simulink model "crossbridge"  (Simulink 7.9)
settings: Solver=ode1  StartTime=0.0  StopTime=dt*klokmax  FixedStep=dt  RelTol=1e-3
PreLoadFcn:
  | %This Model has been adapted from the MATLAB code presented in Hoppensteadt
  | %and Peskin "Modling and Simulation in Medicine and the Life Sciences
  | 
  | %Constants for p(x)
  | p1=4;                       %units: pN
  | GAMMA=0.322;                %units: /nm
  | 
  | %Constants for u
  | alpha=14;                   %probability per unit time for attachment: /s
  | beta=126;                   %probability per unit time for detachment: /s
  | n0=10000;                   %number of crossbridges
  | A=5;                        %displacement of newly attached crossbridge: nm
  | dt=0.01/(alpha+beta);       %duration of time step: s
  | klokmax = 4000;
  | 
  | %number of bins for population density function:
  | nbins=round(sqrt(n0*alpha/(alpha+beta)));
  | 
  | %Model parameters
  | Tstart=14/(alpha+beta);    %time at which motion begins: s
  | V=500;                     %shortening velocity for t>Tstart: nm/s
  | 
  | %All crossbridges are initially detached.
  | a=zeros(1,n0);
  | x0=zeros(1,n0);
undefined symbols (not defined in the file or in its folder): randi
libraries: simulink x2

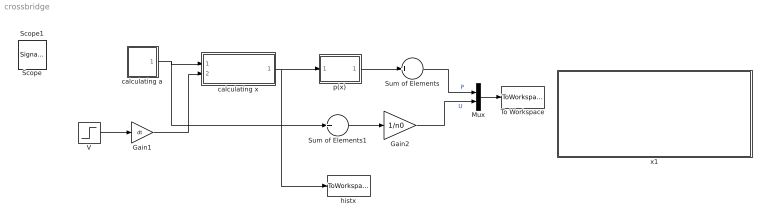
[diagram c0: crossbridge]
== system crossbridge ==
  Gain1 : Gain  Gain=dt
  Gain2 : Gain  Gain=1/n0
  Mux : Mux  Inputs=2
  Sum of Elements : Sum  Inputs=+
  Sum of Elements1 : Sum  Inputs=+
  To Workspace : ToWorkspace  VariableName=P_U  SampleTime=-1  SaveFormat=Structure With Time
  V : Step  Time=Tstart  After=V  SampleTime=0
  calculating a : Subsystem
  calculating x : Subsystem
  histx : ToWorkspace  VariableName=xout  SampleTime=-1
  p(x) : Subsystem
  x1 : Subsystem
  Scope : SignalViewerScope  IOType=viewer  RefreshTime=0.035000
  Scope1 : SignalViewerScope  IOType=viewer  RefreshTime=0.035000
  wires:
  V/1 -> Gain1/1
  calculating a/1(a) -> Sum of Elements1/1, calculating x/1(a)
  Sum of Elements1/1 -> Gain2/1
  Gain1/1 -> calculating x/2(V*dt)
  calculating x/1(calcx) -> histx/1, p(x)/1(calcx)
  Sum of Elements/1 -> Mux/1  "P"
  Gain2/1 -> Mux/2  "U"
  p(x)/1(p) -> Sum of Elements/1
  Mux/1 -> To Workspace/1

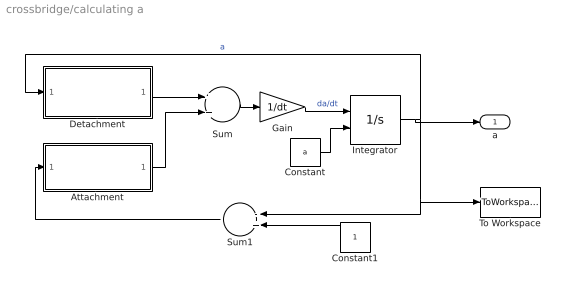
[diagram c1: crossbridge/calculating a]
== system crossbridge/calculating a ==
  Attachment : Subsystem
  Constant : Constant  Value=a
  Constant1 : Constant
  Detachment : Subsystem
  Gain : Gain  Gain=1/dt
  Integrator : Integrator  InitialConditionSource=external
  Sum : Sum
  Sum1 : Sum  Inputs=-+
  To Workspace : ToWorkspace  VariableName=aout  SampleTime=-1
  a : Outport
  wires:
  Integrator/1 -> Detachment/1(a), Sum1/1, To Workspace/1, a/1  "a"
  Constant/1 -> Integrator/2
  Detachment/1(OutD) -> Sum/1
  Attachment/1(OutA) -> Sum/2
  Sum/1 -> Gain/1
  Sum1/1 -> Attachment/1(1-a)
  Constant1/1 -> Sum1/2
  Gain/1 -> Integrator/1  "da/dt"

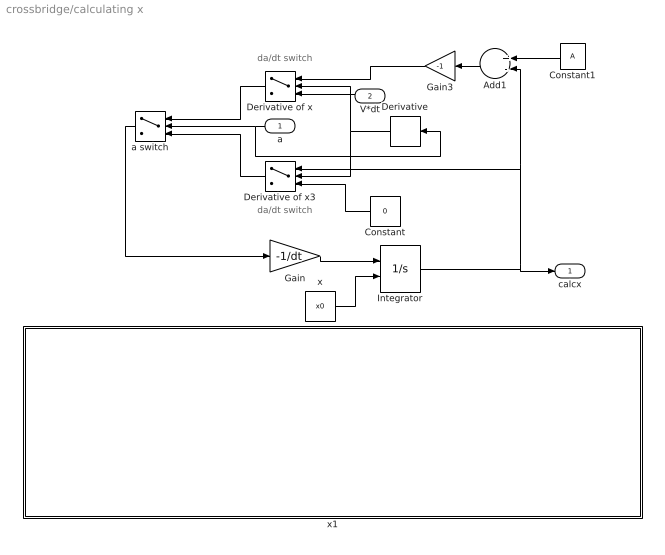
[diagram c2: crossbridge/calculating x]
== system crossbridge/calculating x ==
  note: da/dt switch
  note: da/dt switch
  a : Inport
  V*dt : Inport  Port=2
  Add1 : Sum  Inputs=+-
  Constant : Constant  Value=0
  Constant1 : Constant  Value=A
  Derivative : Derivative
  Derivative of x : Switch  Criteria=u2 ~= 0  ZeroCross=off
  Derivative of x3 : Switch  Criteria=u2 ~= 0  ZeroCross=off
  Gain : Gain  Gain=-1/dt
  Gain3 : Gain  Gain=-1
  Integrator : Integrator  InitialConditionSource=external
  a switch : Switch  Criteria=u2 ~= 0  ZeroCross=off
  x : Constant  Value=x0
  x1 : Subsystem
  calcx : Outport
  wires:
  Gain/1 -> Integrator/1
  Integrator/1 -> calcx/1, Add1/2, Derivative of x3/1
  x/1 -> Integrator/2
  Constant1/1 -> Add1/1
  Add1/1 -> Gain3/1
  Derivative/1 -> Derivative of x3/2, Derivative of x/2
  Derivative of x/1 -> a switch/1
  Derivative of x3/1 -> a switch/3
  a/1 -> a switch/2, Derivative/1
  a switch/1 -> Gain/1
  Constant/1 -> Derivative of x3/3
  V*dt/1 -> Derivative of x/3
  Gain3/1 -> Derivative of x/1

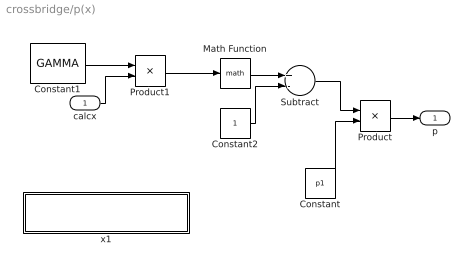
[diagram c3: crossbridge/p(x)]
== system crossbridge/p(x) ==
  calcx : Inport
  Constant : Constant  Value=p1
  Constant1 : Constant  Value=GAMMA
  Constant2 : Constant
  Math Function : Math
  Product : Product
  Product1 : Product
  Subtract : Sum  Inputs=+-
  x1 : Subsystem
  p : Outport
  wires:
  Constant/1 -> Product/2
  Constant1/1 -> Product1/1
  calcx/1 -> Product1/2
  Product1/1 -> Math Function/1
  Math Function/1 -> Subtract/1
  Constant2/1 -> Subtract/2
  Subtract/1 -> Product/1
  Product/1 -> p/1

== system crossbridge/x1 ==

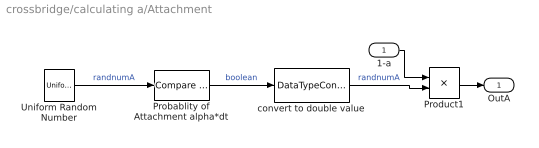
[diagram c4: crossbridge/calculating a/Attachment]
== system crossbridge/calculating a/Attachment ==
  1-a : Inport
  Probablity of Attachment alpha*dt : simulink/Logic and Bit Operations/Compare To Constant  relop=<  const=.001  OutDataTypeStr=boolean  ZeroCross=off
  Product1 : Product
  Uniform Random Number : UniformRandomNumber  Minimum=zeros(1,n0)  Maximum=ones(1,n0)  Seed=randi(n0,[1 n0])  SampleTime=dt
  convert to double value : DataTypeConversion  OutDataTypeStr=double  RndMeth=Ceiling
  OutA : Outport
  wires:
  convert to double value/1 -> Product1/2  "randnumA"
  Probablity of Attachment alpha*dt/1 -> convert to double value/1  "boolean"
  Uniform Random Number/1 -> Probablity of Attachment alpha*dt/1  "randnumA"
  1-a/1 -> Product1/1
  Product1/1 -> OutA/1

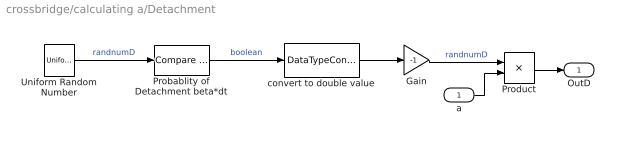
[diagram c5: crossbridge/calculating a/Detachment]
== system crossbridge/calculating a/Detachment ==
  a : Inport
  Gain : Gain  Gain=-1
  Probablity of Detachment beta*dt : simulink/Logic and Bit Operations/Compare To Constant  relop=<  const=.009  OutDataTypeStr=boolean  ZeroCross=off
  Product : Product
  Uniform Random Number : UniformRandomNumber  Minimum=zeros(1,n0)  Maximum=ones(1,n0)  Seed=randi(n0,[1 n0])  SampleTime=dt
  convert to double value : DataTypeConversion  OutDataTypeStr=double  RndMeth=Ceiling
  OutD : Outport
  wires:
  Probablity of Detachment beta*dt/1 -> convert to double value/1  "boolean"
  Uniform Random Number/1 -> Probablity of Detachment beta*dt/1  "randnumD"
  convert to double value/1 -> Gain/1
  Gain/1 -> Product/1  "randnumD"
  a/1 -> Product/2
  Product/1 -> OutD/1

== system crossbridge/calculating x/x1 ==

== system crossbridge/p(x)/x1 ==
